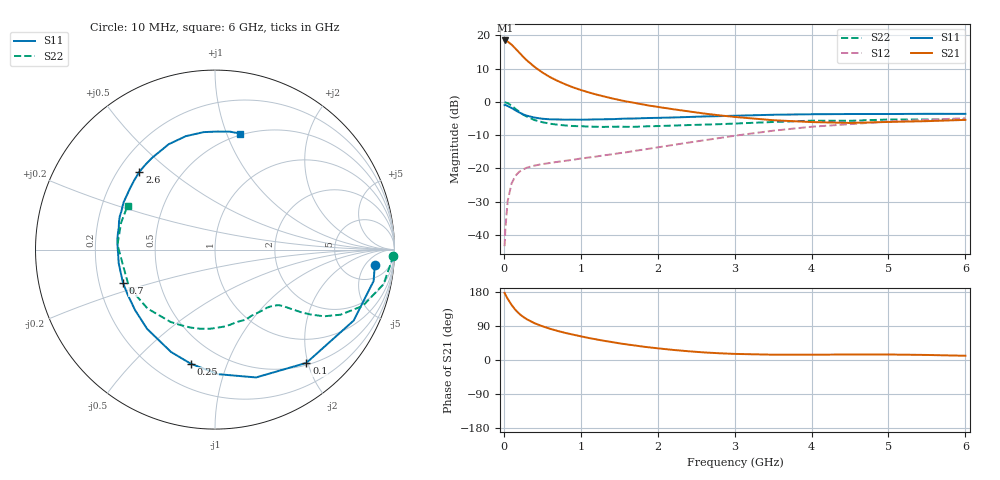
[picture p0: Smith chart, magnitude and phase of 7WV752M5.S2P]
! Infineon Technologies  Discrete & RF Semiconductors
! BFS17W
! Si NPN RF Bipolar Junction Transistor in SOT323
! VCE = 0.75 V  IC = 2.5 mA
! Common Emitter S-Parameters:  August  1999
# GHz  S  MA  R  50
!  f  S11  S21  S12  S22
! GHz  MAG  ANG  MAG  ANG  MAG  ANG  MAG  ANG
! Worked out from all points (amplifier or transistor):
!   36 points, 10 MHz to 6 GHz, reference 50 ohm
!   highest |S21| = 18.5 dB at 20 MHz (marker M1)
!   |S21| within 3 dB of that: start of sweep to 173.9 MHz
!   unconditionally stable (mu >= 1): 675.9 MHz to end of sweep
!   at 250 MHz: K = 0.44, MSG = 16.9 dB, |S12| = -20.3 dB
!   at 1.4 GHz: K = 1.41, MAG = 4.6 dB, |S12| = -15.8 dB
!   at 6 GHz: K = 1.14, MAG = -2.5 dB, |S12| = -4.9 dB
!   S11 on the Smith chart (normalised r, x): 10 MHz: 10, -9; 100 MHz: 0.54, -1.97; 250 MHz: 0.34, -0.75; 700 MHz: 0.30, -0.16; 2.6 GHz: 0.29, +0.39; 6 GHz: 0.49, +1.12
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0.01  0.8944 -5.4  8.347 177.0  0.0068 87.6  0.9949 -1.9
0.02  0.901 -11.2  8.384 172.6  0.0125 85.5  0.9816 -4.7
0.05  0.8678 -27.1  8.065 161.5  0.0325 75.5  0.9586 -11.6
0.1  0.8109 -51.1  7.269 145.6  0.0593 63.3  0.8807 -20.9
0.15  0.7481 -72.2  6.346 132.3  0.0774 53.1  0.788 -27.4
0.2  0.6942 -88.6  5.518 122.1  0.0892 47.4  0.7114 -31.5
0.25  0.6502 -101.9  4.784 114.0  0.0966 42.3  0.6454 -34.1
0.3  0.6209 -113.2  4.202 107.4  0.1029 39.6  0.6006 -35.8
0.4  0.5815 -130.6  3.353 97.0  0.1106 36.2  0.5328 -38.1
0.5  0.5586 -142.8  2.773 89.1  0.1163 35.1  0.4961 -39.5
0.6  0.5476 -152.4  2.36 82.4  0.121 35.1  0.4707 -41.1
0.7  0.5451 -160.1  2.066 76.7  0.1259 35.8  0.4546 -43.3
0.9  0.5418 -172.1  1.654 66.9  0.135 37.7  0.434 -48.3
1.1  0.5429 178.3  1.393 58.2  0.1459 40.1  0.4265 -54.2
1.3  0.5487 170.1  1.21 50.7  0.1577 42.2  0.4211 -61.1
1.6  0.5622 160.6  1.013 41.1  0.1757 45.4  0.4219 -71.4
2.2  0.5837 144.2  0.777 26.6  0.2256 49.5  0.4413 -93.1
2.6  0.6045 134.2  0.67 20.0  0.2648 50.1  0.4556 -107.7
3.5  0.6413 113.7  0.531 14.0  0.3692 45.7  0.4992 -138.9
4.5  0.6576 95.5  0.483 14.5  0.4633 34.9  0.5207 -171.1
5.5  0.6624 82.7  0.514 13.3  0.5381 24.6  0.5442 164.2
6  0.6614 77.8  0.537 11.2  0.5695 19.5  0.545 153.4
